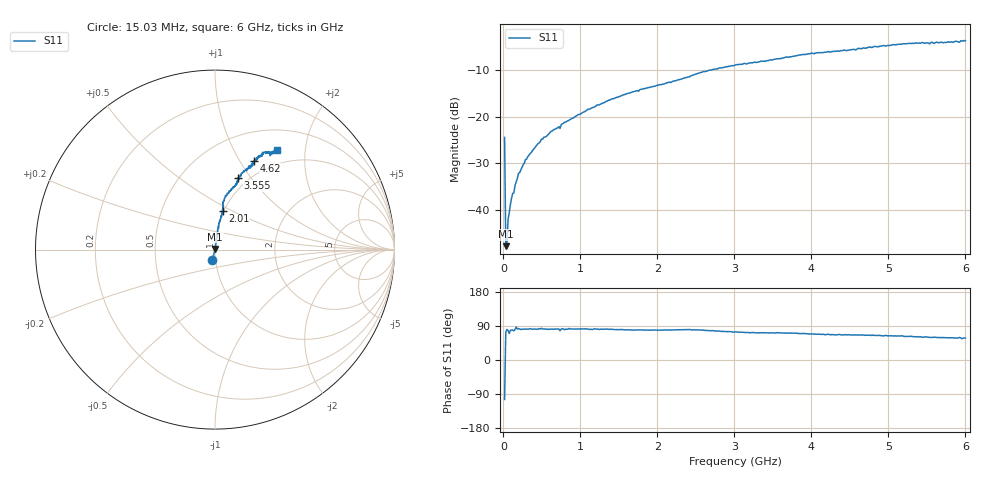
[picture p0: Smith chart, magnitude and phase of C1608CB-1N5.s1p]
!	Network	Analyzer	HP8753E.07.74:	Oct	30	2002	Serial	No.	JP38451487
!	Hewlett-Packard
!	7	Sep	2009	9:29:01
!	Frequency	S11
#	HZ	S	RI	R	50
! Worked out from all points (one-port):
!   400 points, 15.03 MHz to 6 GHz, reference 50 ohm
!   lowest |S11| = -47.8 dB at 30.03 MHz (marker M1), VSWR 1.01, Z = 50.1 + j0.393 ohm
!   |S11| at or under -10 dB: start of sweep to 2.67 GHz
!   S11 on the Smith chart (normalised r, x): 15.03 MHz: 0.96, -0.11; 2.01 GHz: 0.99, +0.44; 3.555 GHz: 0.89, +0.87; 4.62 GHz: 0.83, +1.15; 6 GHz: 0.78, +1.51
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1.502992e7  -0.0145 -0.0583
3.002985e7  0.00119 0.00392
4.502978e7  0.000675 0.00416
6.00297e7  0.00166 0.00777
9.002955e7  0.00231 0.0112
1.200294e8  0.00284 0.0148
1.350293e8  0.00348 0.0149
1.500292e8  0.003 0.0181
1.95029e8  0.00301 0.0245
2.850286e8  0.005 0.0344
4.950275e8  0.00624 0.0576
7.200264e8  0.0111 0.0778
7.350263e8  0.0166 0.0731
7.650262e8  0.0103 0.0836
1.215024e9  0.0193 0.133
1.515022e9  0.0274 0.163
2.01002e9  0.0427 0.214
2.265019e9  0.043 0.245
3.015015e9  0.0983 0.347
3.555012e9  0.127 0.4
3.765011e9  0.145 0.421
4.515007e9  0.216 0.479
4.620007e9  0.218 0.494
5.265004e9  0.286 0.544
5.535002e9  0.307 0.523
5.925e9  0.318 0.544
5.955e9  0.364 0.543
6e9  0.348 0.554
